(* Process data send to or received from IEC 60870-5-101 slave device (LowLevelSlaveSample101 project) *)
TYPE ST_IEC870_5_101MProcData :
STRUCT
	(* Monitoring data points received from IEC 60870-5-101 slave device *)
	stSiq100		: ST_IEC870_5_101SIQ;(* Single point information + quality flags, M_SP_NA_1, IOA = 100 *)
	stSiq101		: ST_IEC870_5_101SIQ;(* Single point information + quality flags, M_SP_TA_1, IOA = 101 *)
	stSiq102		: ST_IEC870_5_101SIQ;(* Single point information + quality flags, M_SP_TB_1, IOA = 102 *)
	
	stDiq200		: ST_IEC870_5_101DIQ;(* Double point information + quality flags, M_DP_NA_1, IOA = 200 *)
	
	nVti300			: BYTE := 0;(* Regulating step value, M_ST_NA_1, IOA = 300 *)
	stQds300		: ST_IEC870_5_101QDS;(* Regulating step quality descriptor *)
	
	nBsi400			: DWORD := 0;(* Bitstring value, M_BO_NA_1, IOA = 400 *)
	stQds400		: ST_IEC870_5_101QDS;(* Bitstring quality descriptor *)
	
	nNva500			: WORD := 0;(* Measured value, normalized value, M_ME_NA_1, IOA = 500 *)
	stQds500		: ST_IEC870_5_101QDS;(* Measured value quality descriptor *)

	nSva600			: INT := 0;(* Mesured value, scaled value, M_ME_NB_1, IOA = 600 *)
	stQds600		: ST_IEC870_5_101QDS;(* Measured value quality descriptor *)

	fSingle700		: REAL := 0.0;(* Measured value, short floating point value, M_ME_NC_1, IOA = 700 *)
	stQds700		: ST_IEC870_5_101QDS;(* Measured value quality descriptor *)
	
	nBcr800			: DINT := 0;(* Binary counter value, M_IT_NA_1, IOA = 800 *)
	nQcr800			: ST_IEC870_5_101QCR;(* Binary counter quality descriptor *)

	nBcr801			: DINT := 0;(* Binary counter value, M_IT_TA_1, IOA = 801 *)
	nQcr801			: ST_IEC870_5_101QCR;(* Binary counter quality descriptor *)

	nBcr802			: DINT := 0;(* Binary counter value, M_IT_TB_1, IOA = 802 *)
	nQcr802			: ST_IEC870_5_101QCR;(* Binary counter quality descriptor *)
	
	(*  Commands send to IEC 60870-5-101 slave device *)
	eScs10			: E_IEC870_5_101SCS := eIEC870_SCS_OFF;(* Single command state, C_SC_NA_1, IOA = 10 *)
	eQu10		 	: E_IEC870_5_101QU := eIEC870_QU_UNSPECIFIED;(* Single command qualifier *)
	eCtrl10 		: E_IEC870_5_101CommandState := eIEC870_CMD_NONE;(* Command exeuction/activation control variable (write eIEC870_CMD_EXECUTE to activate) *)
	
	eDcs20			: E_IEC870_5_101DCS := eIEC870_DCS_OFF;(* Double command state, C_DC_NA_1, IOA = 20 *)
	eQu20			: E_IEC870_5_101QU := eIEC870_QU_UNSPECIFIED;(* Double command qualifier *)
	eCtrl20 		: E_IEC870_5_101CommandState := eIEC870_CMD_NONE;(* Command exeuction/activation control variable (write eIEC870_CMD_EXECUTE to activate) *)
	
	eRcs30			: E_IEC870_5_101RCS := eIEC870_RCS_NOTALLOWED0;(* Regulating step command state, C_RC_NA_1, IOA = 30 *)
	eQu30			: E_IEC870_5_101QU := eIEC870_QU_UNSPECIFIED;(* Regulating step command qualifier *)
	eCtrl30 		: E_IEC870_5_101CommandState := eIEC870_CMD_NONE;(* Command exeuction/activation control variable (write eIEC870_CMD_EXECUTE to activate) *)

	nBsi40			: DWORD := 0;(* Binary state information, C_BO_NA_1, IOA = 40 *)
	eCtrl40 		: E_IEC870_5_101CommandState := eIEC870_CMD_NONE;(* Command exeuction/activation control variable (write eIEC870_CMD_EXECUTE to activate) *)
	
	nNva50			: WORD := 0;(* Setpoint value, normlized value, C_SE_NA_1, IOA = 50 *)
	eQl50			: E_IEC870_5_101QL := eIEC870_QL_DEFAULT;(* Qualifier of setpoint command *)
	eCtrl50 		: E_IEC870_5_101CommandState := eIEC870_CMD_NONE;(* Command exeuction/activation control variable (write eIEC870_CMD_EXECUTE to activate) *)

	nSva60			: INT := 0;(* Setpoint value, scalled value, C_SE_NB_1, IOA = 60 *)
	eQl60			: E_IEC870_5_101QL := eIEC870_QL_DEFAULT;(* Qualifier of setpoint command *)
	eCtrl60 		: E_IEC870_5_101CommandState := eIEC870_CMD_NONE;(* Command exeuction/activation control variable (write eIEC870_CMD_EXECUTE to activate) *)

	fSingle70		: REAL := 0;(* Setpoint value, short floating point value value, C_SE_NC_1, IOA = 70 *)
	eQl70			: E_IEC870_5_101QL := eIEC870_QL_DEFAULT;(* Qualifier of setpoint command *)
	eCtrl70 		: E_IEC870_5_101CommandState := eIEC870_CMD_NONE;(* Command exeuction/activation control variable (write eIEC870_CMD_EXECUTE to activate) *)

END_STRUCT
END_TYPE
